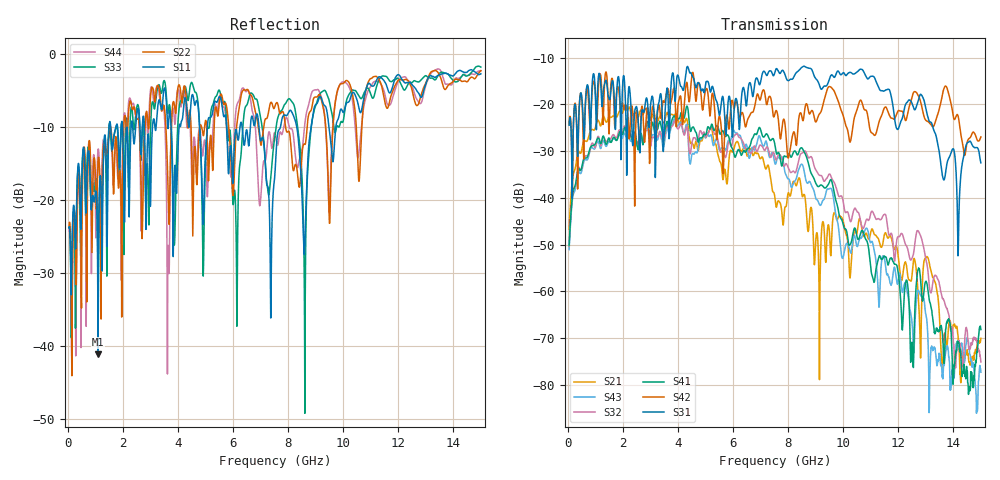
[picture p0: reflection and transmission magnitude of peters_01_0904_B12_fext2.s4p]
# MHZ S RI R 50.00
! FREQ  S11  S12  S13  S14
!  S21  S22  S23  S24
!  S31  S32  S33  S34
!  S41  S42  S43  S44
!  REAL  IMAG  REAL  IMAG  REAL  IMAG  REAL  IMAG
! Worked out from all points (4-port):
!   1496 points, 50 MHz to 15 GHz, reference 50 ohm
!   strongest paths, dB at 50 MHz, 3.79 GHz, 7.53 GHz, 11.27 GHz, 15 GHz:
!     S31: -24.5, -13.6, -13.0, -16.1, -32.5
!     S42: -24.3, -18.5, -21.8, -24.4, -27.0
!     S41: -50.2, -23.3, -28.9, -53.3, -68.2
!     S32: -50.4, -24.7, -31.4, -44.5, -75.1
!     S43: -51.1, -24.4, -32.8, -59.9, -77.3
!     S21: -46.7, -22.2, -40.3, -48.7, -70.1
!   lowest |S11| = -41.2 dB at 1.1 GHz (marker M1), VSWR 1.02, Z = 50.6 + j0.596 ohm
!   |S11| at or under -10 dB: start of sweep to 1.503 GHz; 6.942 GHz to 7.724 GHz (782.8 MHz wide, 10.7 % of centre); 8.313 GHz to 8.84 GHz (527.1 MHz wide, 6.15 % of centre)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
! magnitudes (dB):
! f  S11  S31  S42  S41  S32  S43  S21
! 50 MHz  -23.8  -24.5  -24.3  -50.2  -50.4  -51.1  -46.7
! 1.1 GHz  -41.2  -15.0  -18.2  -27.2  -26.9  -27.9  -23.4
! 8.05 GHz  -7.8  -14.8  -30.5  -30.7  -34.2  -36.2  -39.5
! 8.62 GHz  -24.6  -12.0  -20.6  -30.6  -30.0  -35.5  -40.1
! 9.16 GHz  -5.9  -16.3  -21.9  -37.4  -35.3  -41.6  -58.0
! 12.5 GHz  -4.3  -19.8  -18.5  -70.9  -52.9  -66.8  -56.6
! 15 GHz  -2.8  -32.5  -27.0  -68.2  -75.1  -77.3  -70.1
